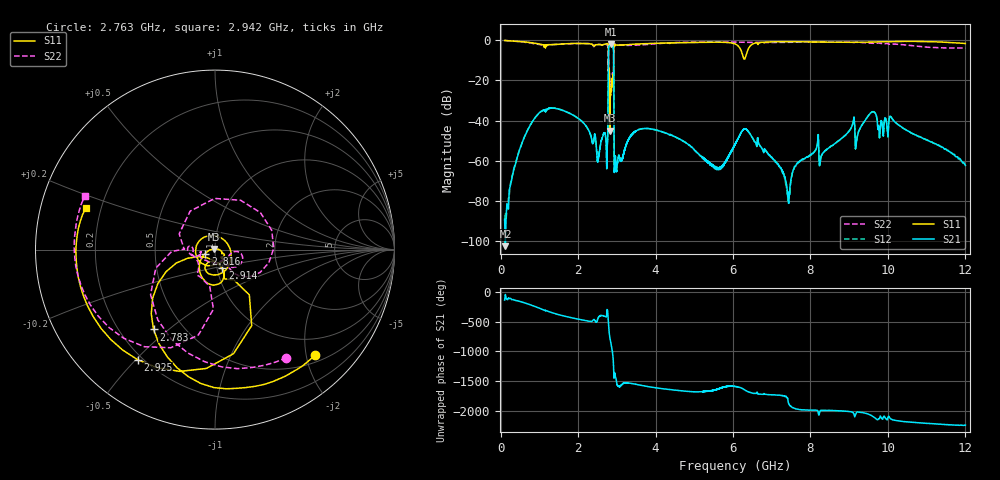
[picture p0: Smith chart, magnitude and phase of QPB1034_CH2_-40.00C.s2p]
! TDS: k:\Engsetup\Winsaw\QPB1034_ALL
! Channel 1
! Ports=1 2
! seg 1=100.000000 1100.000000 51
! seg 2=1101.000000 1301.000000 201
! seg 3=1302.000000 2302.000000 101
! seg 4=2303.000000 3503.000000 1201
! seg 5=3504.000000 5204.000000 171
! seg 6=5205.000000 6405.000000 1201
! seg 7=6406.000000 8506.000000 211
! seg 8=8507.000000 12007.000000 176
! Points=3313
! FailCode=0
! Topology=ALL_SE(12)
!VNA Cal loaded =QPB1034_ALL_-40C
!PS1(V)= 5.000
!PS(mA)= 0.424
!PS2(V)= 0.630
!PS(mA)= -0.001
!PS3(V)= 1.170
!PS(mA)= 0.000
!PS4(V)= 0.630
!PS(mA)= -0.001
!Temp (C)= -40.00
# MHz S DB R 50
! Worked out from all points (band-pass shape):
!   3313 points, 100 MHz to 12.01 GHz, reference 50 ohm
!   highest |S21| = -1.99 dB at 2.844 GHz (marker M1); lowest = -102.4 dB at 120 MHz (marker M2)
!   |S21| within 3 dB of the highest: 2.788 GHz to 2.915 GHz (127 MHz wide, 4.45 % of centre)
!   lowest |S11| = -45.0 dB at 2.822 GHz (marker M3), VSWR 1.01, Z = 49.5 + j0.282 ohm
!   |S11| at or under -10 dB: 2.787 GHz to 2.919 GHz (132.3 MHz wide, 4.64 % of centre)
!   |S22| runs from -23.0 to -0.3 dB; largest |S21 - S12| = 0.0044
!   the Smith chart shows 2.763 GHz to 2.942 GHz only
!   S11 on the Smith chart (normalised r, x): 2.763 GHz: 0.63, -2.18; 2.783 GHz: 0.34, -0.44; 2.816 GHz: 0.90, -0.04; 2.914 GHz: 1.06, -0.22; 2.925 GHz: 0.18, -0.51; 2.942 GHz: 0.14, +0.15
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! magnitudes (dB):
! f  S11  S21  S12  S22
! 100 MHz  -0.3  -89.1  -89.7  -0.3
! 120 MHz  -0.3  -102.4  -85.8  -0.3
! 240 MHz  -0.4  -73.0  -72.9  -0.5
! 500 MHz  -0.8  -53.7  -53.6  -0.8
! 1.1 GHz  -2.5  -35.0  -35.0  -2.6
! 2.434 GHz  -2.6  -47.2  -47.0  -2.6
! 2.506 GHz  -2.3  -60.2  -60.2  -2.3
! 2.74 GHz  -1.9  -63.1  -62.8  -2.2
! 2.763 GHz  -1.8  -49.2  -49.2  -2.8
! 2.783 GHz  -5.0  -9.0  -9.0  -9.5
! 2.816 GHz  -24.6  -2.3  -2.2  -20.8
! 2.822 GHz  -45.0  -2.2  -2.1  -22.8
! 2.844 GHz  -27.2  -2.0  -2.0  -22.2
! 2.914 GHz  -19.2  -4.7  -4.8  -16.8
! 2.925 GHz  -2.5  -38.1  -38.1  -2.5
! 2.942 GHz  -2.5  -64.8  -64.8  -2.1
! 3.774 GHz  -1.8  -43.9  -43.9  -2.3
! 5.406 GHz  -1.1  -61.3  -61.3  -1.0
! 6.321 GHz  -8.8  -44.1  -44.1  -1.2
! 7.436 GHz  -0.9  -81.0  -76.5  -1.2
! 9.647 GHz  -1.0  -35.8  -35.7  -1.7
! 12.01 GHz  -1.8  -62.3  -61.9  -4.0
